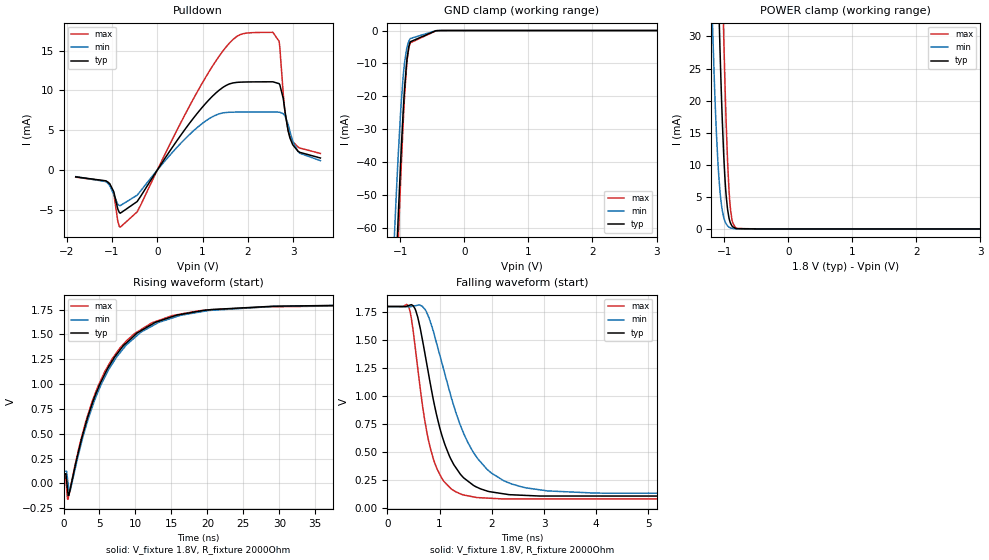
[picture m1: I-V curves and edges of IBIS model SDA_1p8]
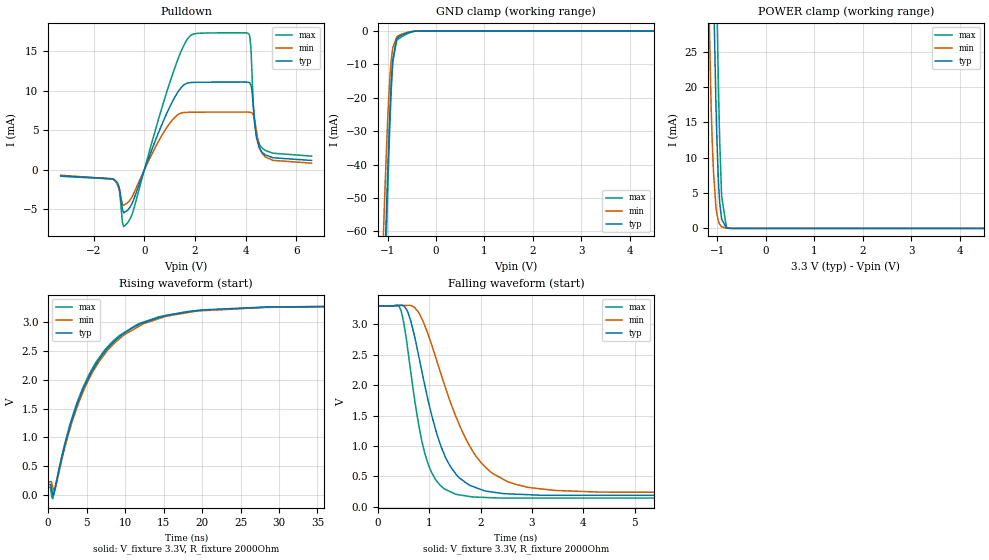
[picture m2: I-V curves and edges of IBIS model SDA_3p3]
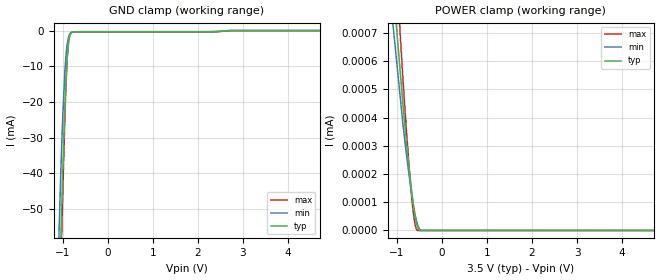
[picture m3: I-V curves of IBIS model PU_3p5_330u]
|Texas Instruments Incorporated
| Marketing part#   Digital Voltage Range   Package-type   #pins
|   TUSB320L   2.7V - 5.0V   X2QFN   12
[IBIS Ver]   4.1
[File name]   tusb320l.ibs
[File Rev]   1.0
[Date]   06/08/2015
[Source]
| Texas Instruments Incorporated.
| 12500 TI Blvd
| Dallas, TX -75243
[Notes]   Revision History:
| Rev 1.0: 06/08/2015
| - Initial version of the model
| - Model generated from simulations in TISPICE
| - C_comp although listed in numerical order of value are
|   obtained from varying PVT conditions. For PVT conditions for
|   each specific value refer the buffer description under
|   respective [Model]. IBIS model user is responsible for using
|   appropriate C_comp to simulate for Signal Integrity.
| - Warnings regarding combined Non-monotonicity of various models have been
|   reviewd and considered minor and can be ignored.
| - Model names with a trailing _2p7 contain the model for
|   2.7V operation. Model names with a trailing _5p0 contain the model
|   for 5.0V operation.
| - CC1 and CC2 pin have a number of models depending pull-up and pull-down
|   cases (pu_xxx_xxx and pd_xxx respectively). Pull-up model also features
|   dependng on the strength of pull up (pu_xxx_80u, pu_xxx_180u and
|   pu_xxx_330u).
[Disclaimer]
| This model is designed as an aid for customers of Texas Instruments.
| TI and its licensors and suppliers make no warranties, either expressed
| or implied, with respect to this  model, including the warranties of
| merchantability or fitness for a particular purpose. The model is
| provided solely on an "as is" basis. The entire risk as to its quality
| and performance is with the customer.
[Copyright]
 (C) Copyright 2015 Texas Instruments Incorporated.All rights reserved.
|   Device
[Component]  TUSB320L
[Manufacturer]   TI
[Package]  |X2QFN   12
|   typ   min   max
R_pkg   0.067   0.027   0.083
L_pkg   0.937nH   0.593nH   1.143nH
C_pkg   0.144pF   0.126pF   0.200pF
[Pin]  signal_name   model_name   R_pin   L_pin   C_pin
1   CC1   CC   NA   NA   NA
2   CC2   CC   NA   NA   NA
3   PORT   ADDR   NA   NA   NA
4   VBUS_DET   NC   NA   NA   NA
5   ADDR   ADDR   NA   NA   NA
6   INT_N/OUT3   INT   NA   NA   NA
7   SDA/OUT1   SDA   NA   NA   NA
8   SCL/OUT2   SDA   NA   NA   NA
9   ID   INT   NA   NA   NA
10   GND   GND   NA   NA   NA
11   EN_N   EN   NA   NA   NA
12   VDD   POWER   NA   NA   NA
|   Model Selectors
[Model Selector]  ADDR
ADDR_5p0  ADDR input buffer at 5.0V operation.
ADDR_2p7  ADDR input buffer at 2.7V operation.
[Model Selector]  EN
EN_5p0  EN input buffer at 5.0V operation.
EN_2p7  EN input buffer at 2.7V operation.
[Model Selector]  INT
INT_5p0  INT buffer at 5.0V operation.
INT_2p7  INT buffer at 2.7V operation.
[Model Selector]  SDA
SDA_3p3  SDA buffer at 3.3V operation.
SDA_1p8  SDA buffer at 1.8V operation.
[Model Selector]  CC
PD_5p0  CC1/CC2 buffer at pull-down state at 5.0V VCC.
PD_2p7  CC1/CC2 buffer at pull-down state at 2.7V VCC.
PU_5p0_80u  CC1/CC2 buffer at 80uA pull-up state at 5.0V VCC.
PU_5p0_180u  CC1/CC2 buffer at 180uA pull-up state at 5.0V VCC.
PU_5p0_330u  CC1/CC2 buffer at 330uA pull-up state at 5.0V VCC.
PU_2p7_80u  CC1/CC2 buffer at 80uA pull-up state at 2.7V VCC.
PU_2p7_180u  CC1/CC2 buffer at 180uA pull-up state at 2.7V VCC.
PU_3p5_330u  CC1/CC2 buffer at 330uA pull-up state at 3.5V VCC.
| Models and submodels in the file (16): SDA_1p8 (I/O_open_drain), SDA_3p3 (I/O_open_drain), PU_3p5_330u (Input), PU_5p0_330u (Input), PU_5p0_180u (Input), PU_5p0_80u (Input), PU_2p7_180u (Input), PU_2p7_80u (Input), PD_5p0 (Input), PD_2p7 (Input), INT_5p0 (Open_drain), INT_2p7 (Open_drain), EN_5p0 (Input), EN_2p7 (Input), ADDR_5p0 (Input), ADDR_2p7 (Input)
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|   Model
[Model]   SDA_1p8
Model_type   I/O_open_drain
Polarity   Non-Inverting
Enable   Active-Low
Vinl = 0.54
Vinh = 1.26
Vmeas = 0.9
Vref = 1.8
Cref = 1pF
Rref = 2000
|   typ   min   max
C_comp   1pF   1pF   1pF
[Voltage Range]   1.8   1.799   1.801
[Temperature Range]   27   105   -40
[Pullup Reference]   1.8   1.799   1.801
[Pulldown Reference]   -0   -0   0
[Power Clamp Reference]   1.8   1.799   1.801
[GND Clamp Reference]   0   0   0
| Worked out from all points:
|   slope of the pulldown table from 0 to 0.27 V, typ, clamps not added: 116 ohm
|   POWER clamp passes 1 mA (typ) near -0.90 V on its own axis
|   falling waveform, V_fixture 1.8V, R_fixture 2000Ohm: 20-80 % time 524ps typ, 753ps min, 365ps max; typ from 1.8 V to 0.097 V
|   rising waveform, V_fixture 1.8V, R_fixture 2000Ohm: 20-80 % time 6.95ns typ, 7.17ns min, 6.72ns max; typ from 0.097 V to 1.8 V
[Pulldown]
|   Voltage   I(typ)   I(min)   I(max)
-1.8V     -861.7uA   -829.5uA   -898.8uA
-1.055V   -1.697mA   -1.903mA   -1.756mA
-817.2mV  -5.43mA    -4.472mA   -7.18mA
-444.6mV  -3.959mA   -3.16mA    -5.26mA
997.2mV   7.919mA    5.873mA    10.98mA
1.575V    10.78mA    7.255mA    15.85mA
1.975V    11.07mA    7.293mA    17.21mA
2.687V    10.86mA    7.273mA    16.18mA
2.817V    7.429mA    6.821mA    7.291mA
2.925V    4.079mA    4.907mA    4.283mA
3.141V    2.229mA    2.119mA    2.769mA
3.6V      1.513mA    1.177mA    2.086mA
[GND Clamp]
|   Voltage   I(typ)   I(min)   I(max)
-1.8V     -477.7mA   -433.3mA   -503.9mA
-1.098V   -88.8mA    -65.47mA   -98.86mA
-1.06V    -70.18mA   -49.29mA   -78.84mA
-1.044V   -62.47mA   -42.77mA   -70.47mA
-1.039V   -59.94mA   -40.67mA   -67.71mA
-1.033V   -57.43mA   -38.6mA    -64.97mA
-984.6mV  -36.2mA    -22.04mA   -41.43mA
-930.6mV  -17.09mA   -9.495mA   -19.33mA
-892.8mV  -8.393mA   -4.912mA   -8.993mA
-844.2mV  -3.427mA   -2.45mA    -3.746mA
-396mV    -22.95uA   -18.2uA    -31.49uA
3.6V      0A         0A         0A
[POWER Clamp]
|   Voltage   I(typ)   I(min)   I(max)
-1.8V     416.5mA    342.1mA    467mA
-1.184V   78.87mA    32.83mA    116mA
-1.125V   51.76mA    15.98mA    84.97mA
-1.082V   34.26mA    8.033mA    63.5mA
-1.066V   28.4mA     5.989mA    55.78mA
-1.033V   18.16mA    3.173mA    41.1mA
-1.006V   11.46mA    1.801mA    29.9mA
-968.4mV  5.192mA    787uA      16.58mA
-919.8mV  1.521mA    263.6uA    5.398mA
-871.2mV  394.5uA    87.13uA    1.15mA
-795.6mV  45.22uA    15.45uA    73.94uA
3.6V      0A         0A         0A
[Ramp]
R_load = 2000
|   typ   min   max
dV/dt_r   1.0217/6.85247e-09   1.00587/7.07089e-09   1.03669/6.69844e-09
dV/dt_f   1.0217/5.23594e-10   1.00587/7.49816e-10   1.03669/3.63608e-10
[Falling Waveform]
V_fixture = 1.8V
V_fixture_min = 1.799V
V_fixture_max = 1.801V
R_fixture = 2000Ohm
C_fixture = 0F
|   Time   V(typ)   V(min)   V(max)
0s        1.8V       1.799V     1.801V
416.9ps   1.81V      1.799V     1.784V
544.7ps   1.761V     1.808V     1.386V
755.7ps   1.281V     1.743V     673.4mV
1.038ns   655.1mV    1.305V     264.8mV
1.272ns   383.6mV    910.5mV    151.4mV
1.531ns   240.2mV    592.2mV    105.5mV
2.202ns   124.2mV    247.3mV    76.92mV
4.106ns   102.7mV    128.6mV    76.88mV
200ns     97.17mV    122.5mV    73.18mV
[Rising Waveform]
V_fixture = 1.8V
V_fixture_min = 1.799V
V_fixture_max = 1.801V
R_fixture = 2000Ohm
C_fixture = 0F
|   Time   V(typ)   V(min)   V(max)
0s        97.17mV    122.5mV    73.18mV
282ps     96.16mV    122mV      72.25mV
579ps     -75.06mV   32.04mV    -161mV
903.1ps   -66.45mV   -77.41mV   -62.75mV
2.342ns   398.2mV    365.7mV    418.3mV
3.979ns   799.8mV    764.9mV    823.7mV
7.798ns   1.337V     1.31V      1.359V
13.22ns   1.632V     1.621V     1.641V
18.71ns   1.732V     1.722V     1.736V
200ns     1.8V       1.799V     1.801V
|   Model
[Model]   SDA_3p3
Model_type   I/O_open_drain
Polarity   Non-Inverting
Enable   Active-Low
Vinl = 0.99
Vinh = 2.31
Vmeas = 1.65
Vref = 3.3
Cref = 1pF
Rref = 2000
|   typ   min   max
C_comp   1pF   1pF   1pF
[Voltage Range]   3.3   3.299   3.301
[Temperature Range]   27   105   -40
[Pullup Reference]   3.3   3.299   3.301
[Pulldown Reference]   0   0   0
[Power Clamp Reference]   3.3   3.299   3.301
[GND Clamp Reference]   0   0   0
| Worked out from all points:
|   slope of the pulldown table from 0 to 0.495 V, typ, clamps not added: 118 ohm
|   GND clamp passes 1 mA (typ) near -0.67 V on its own axis
|   POWER clamp passes 1 mA (typ) near -0.89 V on its own axis
|   falling waveform, V_fixture 3.3V, R_fixture 2000Ohm: 20-80 % time 576ps typ, 865ps min, 386ps max; typ from 3.3 V to 0.179 V
|   rising waveform, V_fixture 3.3V, R_fixture 2000Ohm: 20-80 % time 6.6ns typ, 6.79ns min, 6.46ns max; typ from 0.179 V to 3.3 V
[Pulldown]
|   Voltage   I(typ)   I(min)   I(max)
-3.3V     -775.9uA   -683.3uA   -813uA
-1.152V   -1.313mA   -1.399mA   -1.356mA
-973.5mV  -2.521mA   -2.878mA   -2.699mA
-864.6mV  -5.035mA   -4.366mA   -6.666mA
-676.5mV  -5.168mA   -4.213mA   -6.781mA
1.264V    9.53mA     6.831mA    13.46mA
2.095V    11.08mA    7.296mA    17.27mA
4.125V    11.06mA    7.298mA    17.21mA
4.204V    10.73mA    7.263mA    15.44mA
4.353V    6.01mA     6.378mA    5.868mA
4.541V    2.737mA    2.92mA     3.21mA
6.6V      1.186mA    843.5uA    1.733mA
[GND Clamp]
|   Voltage   I(typ)   I(min)   I(max)
-3.3V     -1.349A    -1.276A    -1.4A
-1.112V   -95.92mA   -71.79mA   -106.5mA
-1.082V   -81.03mA   -58.65mA   -90.53mA
-1.053V   -66.59mA   -46.23mA   -74.95mA
-1.003V   -44mA      -27.89mA   -50.16mA
-973.5mV  -31.79mA   -18.89mA   -36.43mA
-924mV    -15.25mA   -8.461mA   -17.14mA
-894.3mV  -8.65mA    -5.039mA   -9.291mA
-815.1mV  -2.406mA   -1.841mA   -2.897mA
-726mV    -1.369mA   -1.037mA   -1.881mA
-369.6mV  -11.74uA   -10.2uA    -15.01uA
6.6V      0A         0A         0A
[POWER Clamp]
|   Voltage   I(typ)   I(min)   I(max)
-3.3V     1.3A       1.213A     1.36A
-1.221V   96.73mA    46.01mA    135.6mA
-1.132V   54.75mA    17.6mA     88.5mA
-1.082V   34.49mA    8.118mA    63.79mA
-1.013V   13mA       2.086mA    32.65mA
-983.4mV  7.256mA    1.097mA    21.47mA
-973.5mV  5.834mA    881.4uA    18.17mA
-953.7mV  3.655mA    566.6uA    12.4mA
-914.1mV  1.303mA    231.6uA    4.589mA
-815.1mV  79.27uA    24.14uA    151.9uA
-755.7mV  14.3uA     6.184uA    16.83uA
6.6V      0A         0A         0A
[Ramp]
R_load = 2000
|   typ   min   max
dV/dt_r   1.87248/6.60413e-09   1.84301/6.7851e-09   1.89986/6.453e-09
dV/dt_f   1.87248/5.75258e-10   1.84301/8.64854e-10   1.89986/3.83826e-10
[Falling Waveform]
V_fixture = 3.3V
V_fixture_min = 3.299V
V_fixture_max = 3.301V
R_fixture = 2000Ohm
C_fixture = 0F
|   Time   V(typ)   V(min)   V(max)
0s        3.3V       3.299V     3.301V
445ps     3.31V      3.306V     3.231V
643ps     3.039V     3.306V     2.191V
842.7ps   2.277V     3.11V      1.129V
1.115ns   1.295V     2.48V      457.8mV
1.406ns   669.4mV    1.729V     250.6mV
1.756ns   371mV      1.044V     174.8mV
2.388ns   224.9mV    477.6mV    144.8mV
4.354ns   191.1mV    242.2mV    144.7mV
200ns     179.2mV    227.3mV    134.6mV
[Rising Waveform]
V_fixture = 3.3V
V_fixture_min = 3.299V
V_fixture_max = 3.301V
R_fixture = 2000Ohm
C_fixture = 0F
|   Time   V(typ)   V(min)   V(max)
0s        179.2mV    227.3mV    134.6mV
594.6ps   6.248mV    137.6mV    -67.8mV
852.2ps   84.22mV    70.33mV    90.28mV
2.184ns   876.2mV    825.2mV    903.2mV
3.602ns   1.512V     1.461V     1.547V
7.195ns   2.457V     2.42V      2.491V
12.35ns   2.992V     2.971V     3.002V
17.93ns   3.175V     3.163V     3.182V
49.07ns   3.295V     3.293V     3.286V
200ns     3.3V       3.299V     3.301V
|   Model
[Model]   PU_3p5_330u
Model_type   Input
Vinl = 1.05
Vinh = 2.45
|   typ   min   max
C_comp   1pF   1pF   1pF
[Voltage Range]   3.5   3.499   3.501
[Temperature Range]   27   105   -40
[Power Clamp Reference]   3.5   3.499   3.501
[GND Clamp Reference]   0   0   0
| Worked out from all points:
|   GND clamp passes 1 mA (typ) near -0.82 V on its own axis
[GND Clamp]
|   Voltage   I(typ)   I(min)   I(max)
-3.5V     -1.465A    -1.389A    -1.519A
-1.127V   -102.9mA   -77.81mA   -113.9mA
-1.043V   -61.2mA    -41.4mA    -69.12mA
-1.032V   -56.28mA   -37.33mA   -63.75mA
-1.022V   -51.45mA   -33.39mA   -58.46mA
-1.012V   -46.73mA   -29.62mA   -53.24mA
-990.5mV  -37.65mA   -22.65mA   -43.12mA
-948.5mV  -21.5mA    -11.48mA   -24.6mA
-906.5mV  -9.498mA   -4.724mA   -10.19mA
-864.5mV  -3.086mA   -1.732mA   -2.644mA
-801.5mV  -618.3uA   -520.7uA   -503.5uA
7V        0A         0A         0A
[POWER Clamp]
|   Voltage   I(typ)   I(min)   I(max)
-3.5V     5.553uA    1.275mA    7.545uA
-3.059V   4.68uA     3.893uA    6.352uA
-864.5mV  452.9nA    381.7nA    545.2nA
-749mV    259.8nA    225.7nA    278.8nA
-707mV    195.2nA    173.8nA    191.3nA
-665mV    135.6nA    125.9nA    113.7nA
-633.5mV  95.61nA    93.52nA    65.69nA
-602mV    61.17nA    64.95nA    30.2nA
-570.5mV  33.83nA    41.04nA    8.968nA
-539mV    14.62nA    22.46nA    0A
-476mV    0A         0A         0A
7V        0A         0A         0A
